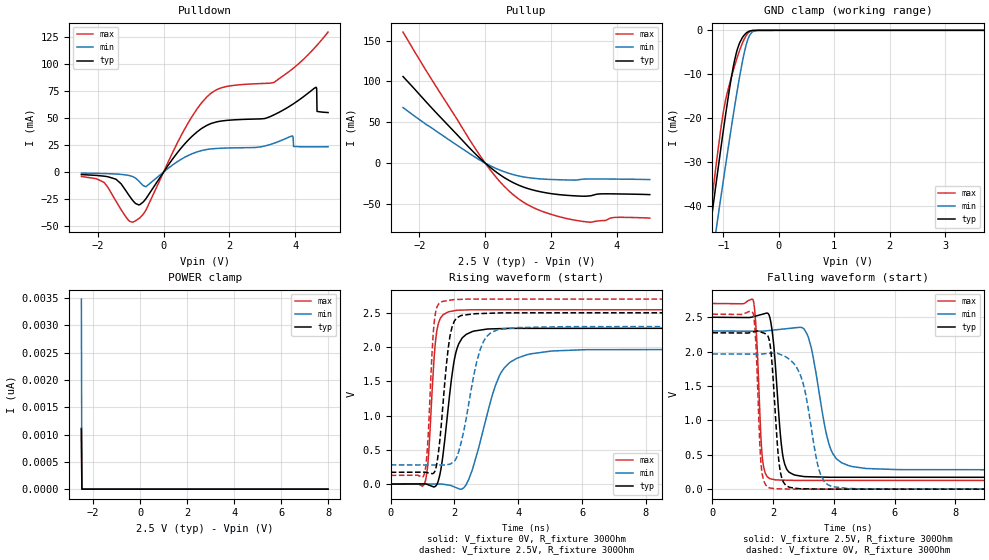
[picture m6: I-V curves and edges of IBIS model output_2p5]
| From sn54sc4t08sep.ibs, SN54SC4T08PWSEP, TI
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|   output_2p5 Model
[Model]   output_2p5
Model_type   3-state
Polarity   Non-Inverting
Vmeas = 1.25
Vref = 0
Cref = 2pF
Rref = 100000
|   typ   min   max
C_comp   5.7pF   5.6pF   6pF
[Voltage Range]   2.5   2.3   2.7
[Temperature Range]   25   125   -40
[Pullup Reference]   2.5   2.3   2.7
[Pulldown Reference]   0   0   0
[Power Clamp Reference]   2.5   2.3   2.7
[GND Clamp Reference]   0   0   0
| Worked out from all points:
|   slope of the pulldown table from 0 to 0.375 V, typ, clamps not added: 23.2 ohm
|   slope of the pullup table from 0 to 0.375 V, typ, clamps not added: 30.9 ohm
|   GND clamp passes 1 mA (typ) near -0.62 V on its own axis
|   falling waveform, V_fixture 2.5V, R_fixture 300Ohm: 20-80 % time 242ps typ, 494ps min, 154ps max; typ from 2.5 V to 0.172 V
|   rising waveform, V_fixture 0V, R_fixture 300Ohm: 20-80 % time 350ps typ, 726ps min, 197ps max; typ from 0 V to 2.27 V
|   rising waveform, V_fixture 2.5V, R_fixture 300Ohm: 20-80 % time 279ps typ, 517ps min, 165ps max; typ from 0.172 V to 2.5 V
|   falling waveform, V_fixture 0V, R_fixture 300Ohm: 20-80 % time 213ps typ, 484ps min, 139ps max; typ from 2.27 V to 0 V
[Pulldown]
|   Voltage   I(typ)   I(min)   I(max)
-2.5V     -2.378mA   -991.6uA   -4.146mA
-1.817V   -3.822mA   -1.402mA   -9.499mA
-1.45V    -6.737mA   -1.857mA   -26.92mA
-851.5mV  -29.25mA   -5.725mA   -45.22mA
-536.5mV  -24.72mA   -13.61mA   -35.32mA
576.5mV   23.84mA    12.59mA    36.38mA
1.312V    43.26mA    20.9mA     69.62mA
3.359V    53.15mA    26.75mA    83.32mA
4.63V     78.6mA     23.38mA    116.6mA
4.651V    77.42mA    23.38mA    117.3mA
4.661V    56.26mA    23.38mA    117.7mA
4.997V    55.19mA    23.48mA    129.9mA
[GND Clamp]
|   Voltage   I(typ)   I(min)   I(max)
-2.5V     -170.7mA   -168.9mA   -187.4mA
-1.282V   -49.09mA   -58.54mA   -46.61mA
-1.24V    -45.04mA   -54.83mA   -42.02mA
-1.208V   -42.02mA   -52.06mA   -38.61mA
-1.125V   -34.05mA   -44.71mA   -29.82mA
-977.5mV  -20.62mA   -32.07mA   -16.86mA
-799mV    -6.847mA   -17.4mA    -8.124mA
-715mV    -3.091mA   -11.05mA   -4.817mA
-641.5mV  -1.357mA   -6.134mA   -2.454mA
-526mV    -161.3uA   -1.092mA   -287.1uA
-379mV    -1.458uA   -24.14uA   -787.4nA
8V        0A         0A         0A
[Pullup]
|   Voltage   I(typ)   I(min)   I(max)
-2.5V     106mA      68.04mA    160.3mA
-1.66V    68.95mA    43.96mA    104.3mA
-169mV    6.211mA    3.858mA    9.77mA
429.5mV   -13.68mA   -8.203mA   -21.93mA
1.018V    -26.96mA   -15.63mA   -43.86mA
1.312V    -31.25mA   -17.72mA   -51.35mA
1.763V    -35.63mA   -19.46mA   -59.38mA
2.897V    -40.29mA   -19.88mA   -70.84mA
3.223V    -39.68mA   -19.28mA   -72.13mA
3.422V    -37.77mA   -19.31mA   -70.64mA
3.958V    -37.57mA   -19.48mA   -66.29mA
4.997V    -38.45mA   -20.07mA   -67.13mA
[POWER Clamp]
|   Voltage   I(typ)   I(min)   I(max)
-2.5V     1.103nA    3.484nA    1.124nA
-2.479V   0A         0A         0A
-2.469V   0A         0A         0A
8V        0A         0A         0A
[Ramp]
R_load = 300
|   typ   min   max
dV/dt_r   1.36436/3.49425e-10   1.17958/7.22573e-10   1.52665/1.95674e-10
dV/dt_f   1.39688/2.41196e-10   1.21189/4.91811e-10   1.544/1.53515e-10
[Falling Waveform]
V_fixture = 2.5V
V_fixture_min = 2.3V
V_fixture_max = 2.7V
R_fixture = 300Ohm
C_fixture = 0F
|   Time   V(typ)   V(min)   V(max)
0s        2.5V       2.3V       2.7V
1.344ns   2.507V     2.297V     2.747V
1.642ns   2.543V     2.296V     473.5mV
1.883ns   2.508V     2.308V     155.2mV
2.307ns   523mV      2.327V     132mV
2.661ns   213.6mV    2.344V     127.9mV
3.143ns   181.1mV    2.226V     127.2mV
3.831ns   173.3mV    666.7mV    127.1mV
4.466ns   173mV      345.5mV    127.1mV
15ns      171.9mV    280.2mV    126.7mV
[Rising Waveform]
V_fixture = 0V
V_fixture_min = 0V
V_fixture_max = 0V
R_fixture = 300Ohm
C_fixture = 0F
|   Time   V(typ)   V(min)   V(max)
0s        1.139uV    -1.683uV   2.742uV
1.071ns   2.549mV    342.2uV    23.54mV
1.178ns   -10.94mV   376.5uV    367.7mV
1.434ns   -14.41mV   458.8uV    2.195V
1.798ns   1.091V     -13.36mV   2.511V
2.002ns   1.832V     -43.15mV   2.53V
2.251ns   2.138V     -66.37mV   2.54V
3.403ns   2.268V     1.575V     2.543V
4.254ns   2.272V     1.885V     2.544V
15ns      2.274V     1.966V     2.544V
[Rising Waveform]
V_fixture = 2.5V
V_fixture_min = 2.3V
V_fixture_max = 2.7V
R_fixture = 300Ohm
C_fixture = 0F
|   Time   V(typ)   V(min)   V(max)
0s        171.9mV    280.2mV    126.7mV
1.053ns   173.7mV    278.7mV    145.5mV
1.159ns   165.5mV    278.6mV    582.3mV
1.36ns    168.1mV    278.3mV    2.34V
1.611ns   1.006V     277.9mV    2.663V
1.802ns   1.975V     286.2mV    2.679V
1.992ns   2.375V     333.5mV    2.693V
2.79ns    2.488V     1.939V     2.7V
3.335ns   2.497V     2.249V     2.7V
15ns      2.5V       2.3V       2.7V
[Falling Waveform]
|Gnd
V_fixture = 0V
V_fixture_min = 0V
V_fixture_max = 0V
R_fixture = 300Ohm
C_fixture = 0F
|   Time   V(typ)   V(min)   V(max)
0s        2.274V     1.966V     2.544V
1.338ns   2.286V     1.964V     2.56V
1.434ns   2.296V     1.964V     2.096V
1.602ns   2.284V     1.965V     368.5mV
1.844ns   2.21V      1.973V     24.09mV
2.217ns   307.8mV    1.963V     4.43mV
2.522ns   29.65mV    1.893V     1.77mV
3.521ns   1.713mV    268.1mV    458.1uV
3.921ns   920uV      41.73mV    442.3uV
15ns      1.377uV    -1.741uV   2.824uV
